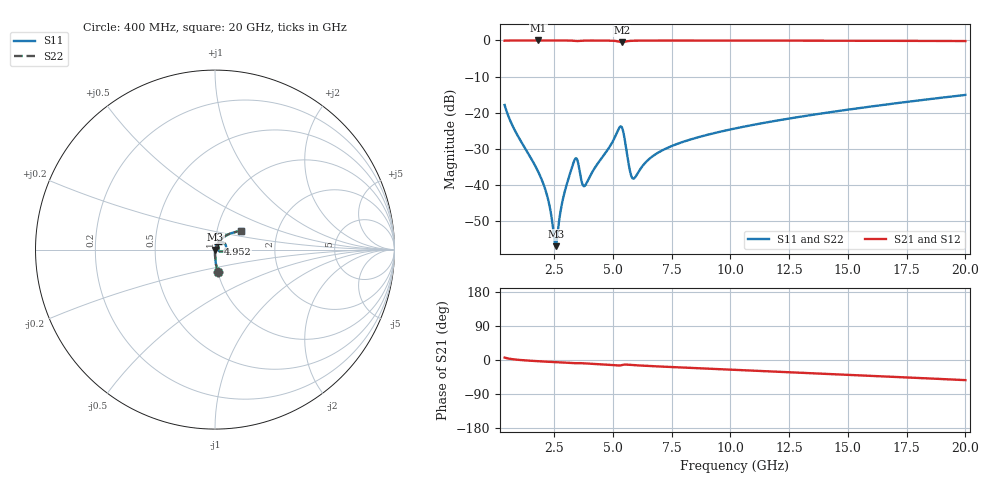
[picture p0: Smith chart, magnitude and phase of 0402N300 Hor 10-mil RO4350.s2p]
# GHz S MA R 50
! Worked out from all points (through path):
!   1960 points, 400 MHz to 20 GHz, reference 50 ohm
!   highest |S21| = -0.01 dB at 1.831 GHz (marker M1); lowest = -0.5 dB at 5.393 GHz (marker M2)
!   group delay of S21, straight-line fit = 7.63 ps
!   lowest |S11| = -56.9 dB at 2.571 GHz (marker M3), VSWR 1.00, Z = 50.1 - j0.0202 ohm
!   |S11| at or under -10 dB: start of sweep to end of sweep
!   |S22| runs from -56.9 to -15.1 dB; largest |S21 - S12| = 0
!   S11 on the Smith chart (normalised r, x): 400 MHz: 1.00, -0.26; 4.952 GHz: 1.03, +0.07; 20 GHz: 1.30, +0.28
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0.4  0.1277 -83.3  0.9913 6.4  0.9913 6.4  0.1277 -83.3
0.8402246  0.05655 -87.9  0.9976 1.4  0.9976 1.4  0.05655 -87.9
1.83073  0.01521 -89.3  0.9988 -3.2  0.9988 -3.2  0.01521 -89.3
2.230934  0.006679 -84.3  0.9987 -4.6  0.9987 -4.6  0.006679 -84.3
2.511077  0.001817 -46.6  0.9985 -5.5  0.9985 -5.5  0.001817 -46.6
2.571108  0.001425 -8.1  0.9985 -5.7  0.9985 -5.7  0.001425 -8.1
2.631138  0.001841 30.1  0.9984 -5.9  0.9984 -5.9  0.001841 30.1
2.911281  0.007046 65.9  0.9978 -6.9  0.9978 -6.9  0.007046 65.9
3.341501  0.02082 50.9  0.9891 -8.5  0.9891 -8.5  0.02082 50.9
3.481572  0.02264 23.2  0.9805 -8.4  0.9805 -8.4  0.02264 23.2
3.671669  0.01137 13.9  0.9893 -8.4  0.9893 -8.4  0.01137 13.9
3.841756  0.01004 45.4  0.994 -9.0  0.994 -9.0  0.01004 45.4
4.952323  0.03758 63.9  0.9907 -13.1  0.9907 -13.1  0.03758 63.9
5.272486  0.06145 37.3  0.9606 -14.5  0.9606 -14.5  0.06145 37.3
5.392547  0.06223 9.1  0.942 -13.3  0.942 -13.3  0.06223 9.1
5.732721  0.01562 -8.8  0.9842 -12.8  0.9842 -12.8  0.01562 -8.8
5.862787  0.01226 19.0  0.9894 -13.4  0.9894 -13.4  0.01226 19.0
6.943338  0.02819 66.1  0.9959 -17.0  0.9959 -17.0  0.02819 66.1
10.205  0.06058 61.5  0.995 -26.0  0.995 -26.0  0.06058 61.5
13.46667  0.09314 53.4  0.9922 -34.8  0.9922 -34.8  0.09314 53.4
16.73834  0.1312 44.7  0.9874 -43.9  0.9874 -43.9  0.1312 44.7
20  0.1762 35.7  0.98 -53.1  0.98 -53.1  0.1762 35.7
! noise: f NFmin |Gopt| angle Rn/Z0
0.4  0.001203  0.7766  1.129  0.001102
2.571  0.005001  0.6747  5.728  0.002957
4.752  0.01285  0.7554  10.5  0.01053
6.933  0.01265  0.6592  15.23  0.006972
9.104  0.01308  0.5882  19.7  0.00565
11.29  0.01478  0.5599  24.12  0.005788
13.47  0.01663  0.5427  28.44  0.006103
15.64  0.0185  0.5314  32.63  0.006464
17.82  0.0204  0.524  36.71  0.006848
20  0.02233  0.5197  40.67  0.00725
